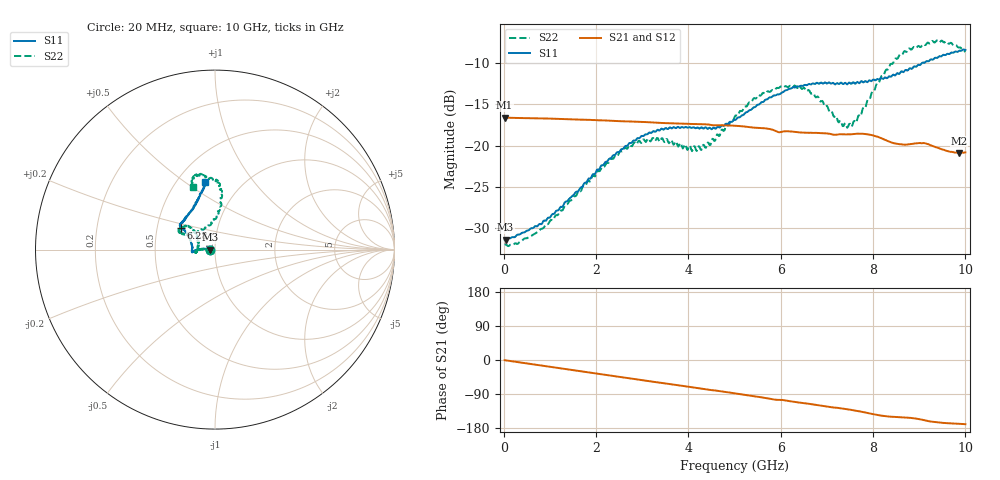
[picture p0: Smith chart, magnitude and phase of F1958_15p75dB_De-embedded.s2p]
! Integrated Device Technology
! Corporate Headquarters
! 6024 Silver Creek Valley Road
! San Jose, CA 95138  USA
! Phone:  1-408-284-8200
! Toll Free:  1-800-223-1366
! Webpage:  http://www.idt.com/
! Timing and RF Division
! 515 Groton Road, Suite 102
! Westford, MA 01886-6024
! Device:  F1958
! Description: 7-bit 0.25 dB Digital Step Attenuator
! Frequency:  0.001 -  6.000 GHz
! Package:  4x4 mm Thin QFN Plastic Package: 24 pin
! Ports:  2 RF, 12 DC
!  Pin  1  = D0
!  Pin  2  = VDD
!  Pin  3  = VMODE
!  Pin  4  = GND
!  Pin  5  = RF1  =  Port 1
!  Pin  6  = GND
!  Pin  7  = GND
!  Pin  8  = GND
!  Pin  9  = GND
!  Pin 10  = GND
!  Pin 11  = GND
!  Pin 12  = GND
!  Pin 13  = GND
!  Pin 14  = RF2  =  Port 2
!  Pin 15  = GND
!  Pin 16  = LE
!  Pin 17  = CLK
!  Pin 18  = DATA
!  Pin 19  = D6
!  Pin 20  = D5
!  Pin 21  = D4
!  Pin 22  = D3
!  Pin 23  = D2
!  Pin 24  = D1
! State:  63
! Atten State:  15.75 dB
! Voltage:  +3.30 Volts
! Current:  0.258 mA
! Data:  The device was measured on a F1958 evaluation board which has
!  individual transmission lines to the RF pins.  Data was collected
!  using a calibrated network analyzer.  The evaluation board was
!  de-embedded using Automatic Fixture Removal (AFR).
!  The reference plane is the edge of the package pin.
! Misc:
!  Action Tracker AT0419
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# GHz S dB R 50
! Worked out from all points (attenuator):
!   500 points, 20 MHz to 10 GHz, reference 50 ohm
!   highest |S21| = -16.61 dB at 20 MHz (marker M1); lowest = -20.9 dB at 9.86 GHz (marker M2)
!   lowest |S11| = -31.4 dB at 40 MHz (marker M3), VSWR 1.06, Z = 47.4 - j0.0708 ohm
!   |S11| at or under -10 dB: start of sweep to 9.059 GHz
!   |S22| runs from -32.2 to -7.3 dB; largest |S21 - S12| = 0.00049
!   S11 on the Smith chart (normalised r, x): 20 MHz: 0.95, -0.00; 6.28 GHz: 0.66, +0.17; 10 GHz: 0.68, +0.60
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0.02  -31.36 -178.4  -16.61 -0.5  -16.60 -0.5  -31.99 -178.5
0.04  -31.38 -178.4  -16.61 -0.8  -16.61 -0.8  -31.94 -177.8
0.32  -30.75 177.1  -16.66 -5.9  -16.66 -5.9  -31.80 177.8
0.84  -29.33 175.0  -16.71 -15.2  -16.70 -15.2  -30.03 178.2
1.7  -25.00 176.0  -16.86 -30.3  -16.85 -30.3  -25.11 177.0
2.6  -20.31 -179.8  -17.06 -46.1  -17.04 -46.2  -20.49 -178.1
2.92  -19.08 -176.8  -17.12 -51.8  -17.10 -51.8  -19.41 -174.7
3.36  -18.16 -174.1  -17.24 -59.5  -17.24 -59.6  -19.36 -170.5
4.24  -17.95 -178.9  -17.40 -74.6  -17.41 -74.6  -20.11 167.4
4.5  -18.02 175.3  -17.52 -79.4  -17.52 -79.5  -19.51 152.0
5.02  -16.89 160.8  -17.59 -88.3  -17.60 -88.3  -16.36 138.7
5.56  -14.87 150.2  -17.87 -98.0  -17.88 -98.0  -13.96 139.8
6.28  -12.94 147.3  -18.32 -110.2  -18.34 -110.2  -12.83 150.7
6.68  -12.51 145.2  -18.45 -116.8  -18.47 -116.7  -13.69 153.4
7.3  -12.38 139.2  -18.62 -127.5  -18.63 -127.4  -17.00 132.6
7.5  -12.41 136.5  -18.63 -131.0  -18.63 -130.9  -17.35 114.5
7.68  -12.37 133.5  -18.55 -134.7  -18.55 -134.7  -16.39 97.7
8.34  -11.63 117.6  -19.49 -149.3  -19.49 -149.4  -10.64 82.5
8.68  -10.98 111.0  -19.89 -151.7  -19.87 -151.6  -8.55 86.9
9.26  -9.55 103.1  -19.98 -162.5  -19.98 -162.5  -7.46 99.5
9.86  -8.54 98.4  -20.88 -168.2  -20.90 -168.1  -8.14 108.4
10  -8.41 98.4  -20.81 -169.4  -20.85 -169.3  -8.65 109.2
